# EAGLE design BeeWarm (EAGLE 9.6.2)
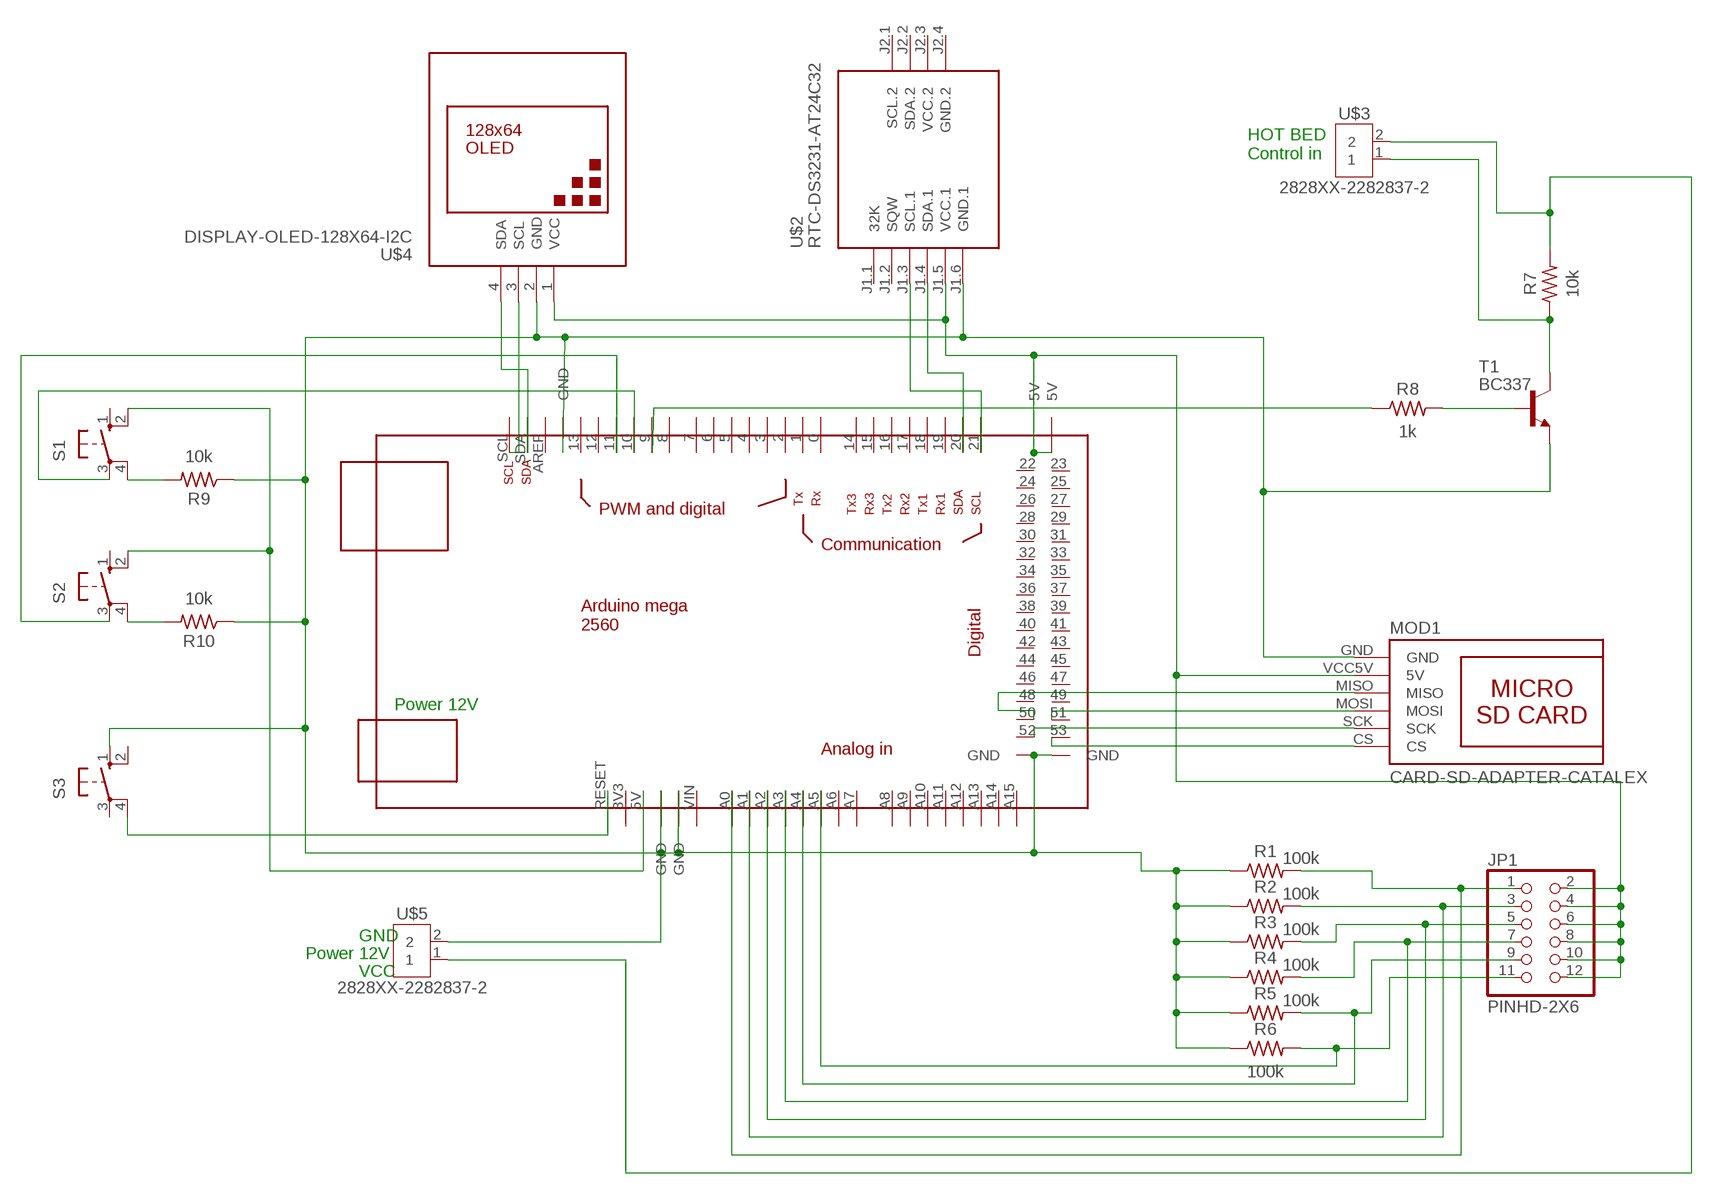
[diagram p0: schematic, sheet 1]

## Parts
JP1  PINHD-2X6  [2X06]
MOD1  CARD-SD-ADAPTER-CATALEX  [CARD-SD-ADAPTER-CATALEX]
R1  100k  R-US_AXIAL-11.7MM-PITCH  [RESAD1176W63L850D250B]
R2  100k  R-US_AXIAL-11.7MM-PITCH  [RESAD1176W63L850D250B]
R3  100k  R-US_AXIAL-11.7MM-PITCH  [RESAD1176W63L850D250B]
R4  100k  R-US_AXIAL-11.7MM-PITCH  [RESAD1176W63L850D250B]
R5  100k  R-US_AXIAL-11.7MM-PITCH  [RESAD1176W63L850D250B]
R6  100k  R-US_AXIAL-11.7MM-PITCH  [RESAD1176W63L850D250B]
R7  10k  R-US_AXIAL-11.7MM-PITCH  [RESAD1176W63L850D250B]
R8  1k  R-US_AXIAL-11.7MM-PITCH  [RESAD1176W63L850D250B]
R9  10k  R-US_AXIAL-11.7MM-PITCH  [RESAD1176W63L850D250B]
R10  10k  R-US_AXIAL-11.7MM-PITCH  [RESAD1176W63L850D250B]
S1  10-XX  [B3F-10XX]
S2  10-XX  [B3F-10XX]
S3  10-XX  [B3F-10XX]
T1  BC337  [TO92]
U$1  MEGA_DEVICE  [MEGAOUTLINE]
U$2  RTC-DS3231-AT24C32  [RTC-DS3231-AT24C32]
U$3  2828XX-2282837-2  [TERMBLK_508-2N]
U$4  DISPLAY-OLED-128X64-I2C  [DISPLAY-OLED-128X64-I2C]
U$5  2828XX-2282837-2  [TERMBLK_508-2N]

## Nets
N$2: S3.4(P1) U$1.RESET
N$3: MOD1.GND R1.1 R2.1 R3.1 R4.1 R5.1 R6.1 R9.1 R10.1 S3.1(S) T1.1(E) U$1.GND@1(GND) U$1.GND@2(GND) U$1.GND@3(GND) U$1.GND@6(GND) U$1.GND@7(GND) U$2.J1.6(GND.1) U$4.2(GND) U$5.2
N$5: JP1.1 R1.2 U$1.A0
N$6: JP1.3 R2.2 U$1.A1
N$7: JP1.5 R3.2 U$1.A2
N$8: JP1.7 R4.2 U$1.A3
N$9: JP1.9 R5.2 U$1.A4
N$10: JP1.11 R6.2 U$1.A5
N$11: U$1.20 U$2.J1.4(SDA.1)
N$12: U$1.21 U$2.J1.3(SCL.1)
N$13: U$1.SDA U$4.4(SDA)
N$14: MOD1.MOSI U$1.51
N$15: MOD1.SCK U$1.52
N$16: MOD1.CS U$1.53
N$17: MOD1.MISO U$1.50
N$18: U$1.SCL U$4.3(SCL)
N$19: R8.2 T1.2(B)
N$20: R7.1 T1.3(C) U$3.1
N$21: R7.2 U$3.2 U$5.1
N$22: R9.2 S1.4(P1)
N$23: R8.1 U$1.9
N$24: R10.2 S2.4(P1)
N$25: S1.3(P) U$1.10
N$26: S2.3(P) U$1.11
N$27: S1.2(S1) S2.2(S1) U$1.5V
N$29: JP1.2 JP1.4 JP1.6 JP1.8 JP1.10 JP1.12 MOD1.VCC5V(5V) U$1.GND@4(5V) U$1.GND@5(5V) U$2.J1.5(VCC.1) U$4.1(VCC)
Unconnected: S1.1(S) S2.1(S) S3.2(S1) S3.3(P) U$1.0 U$1.1 U$1.2 U$1.3 U$1.3V3 U$1.4 U$1.5 U$1.6 U$1.7 U$1.8 U$1.12 U$1.13 U$1.14 U$1.15 U$1.16 U$1.17 U$1.18 U$1.19 U$1.22 U$1.23 U$1.24 U$1.25 U$1.26 U$1.27 U$1.28 U$1.29 U$1.30 U$1.31 U$1.32 U$1.33 U$1.34 U$1.35 U$1.36 U$1.37 U$1.38 U$1.39 U$1.40 U$1.41 U$1.42 U$1.43 U$1.44 U$1.45 U$1.46 U$1.47 U$1.48 U$1.49 U$1.A6 U$1.A7 U$1.A8 U$1.A9 U$1.A10 U$1.A11 U$1.A12 U$1.A13 U$1.A14 U$1.A15 U$1.AREF U$1.VIN U$2.J1.1(32K) U$2.J1.2(SQW) U$2.J2.1(SCL.2) U$2.J2.2(SDA.2)

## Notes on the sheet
- HOT BED 
  Control in
- Power 12V
- GND
- Power 12V
- VCC

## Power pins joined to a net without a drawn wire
GND.2: U$2.J2.4(GND.2)
VCC.2: U$2.J2.3(VCC.2)

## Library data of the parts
JP1 = Connector:PINHD-2X6: PIN HEADER; CATEGORY: CONNECTOR; SUB-CATEGORY: PIN-HEADER
MOD1 = SD-Card-Module_CATALEX:CARD-SD-ADAPTER-CATALEX: Micro SD Card Adapter Module with onboard 3.3V regulator
R1-R10 = Resistor:R-US: Resistor Fixed - ANSI; CATEGORY: Resistor; SUB-CATEGORY: Fixed
S1-S3 = switch-omron:10-XX: OMRON SWITCH; MPN: B3F-1000; OC_FARNELL: 176432; OC_NEWARK: 36M3542
T1 = transistor:BC337: NPN TRANSISTOR
U$1 = ArduinoMegaOutline:MEGA_DEVICE: mega card as device
U$2 = diy-modules:RTC-DS3231-AT24C32: RTC Module with Battery and EEPROM based on DS3231 and AT24C32 chips Tutorial can be found here: https://edwardmallon.wordpress.com/2014/05/21/using-a-cheap-3-ds3231-rtc-at24c32-eeprom-from-ebay/ Click here to find device on ebay.com
U$3 U$5 = Connector:2828XX-2: 2 Position Wire to Board Terminal Block Horizontal with Board; CATEGORY: Connector; DESCRIPTION: 2 Position Wire to Board Terminal Block Horizontal with Board 5.08 mm Through Hole; MANUFACTURER: TE Connectivity; MPN: 282837-2; OPERATING_TEMPERATURE: -40°C to +105°C; PART_STATUS: ACTIVE; ROHS_COMPLIANCE: RoHS Compliant; SERIES: 282837; SUBCATEGORY: Terminal Block; TYPE: Side Wire Entry
U$4 = diy-modules (1):DISPLAY-OLED-128X64-I2C: 128x64 Dot Matrix OLED Module based on SSD1306 chip Variant with I2C interface More details available here: http://www.instructables.com/id/Monochrome-096-i2c-OLED-display-with-arduino-SSD13/ SSD1306 datasheet: https://cdn-shop.adafruit.com/datasheets/SSD1306.pdf Click here to find device on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

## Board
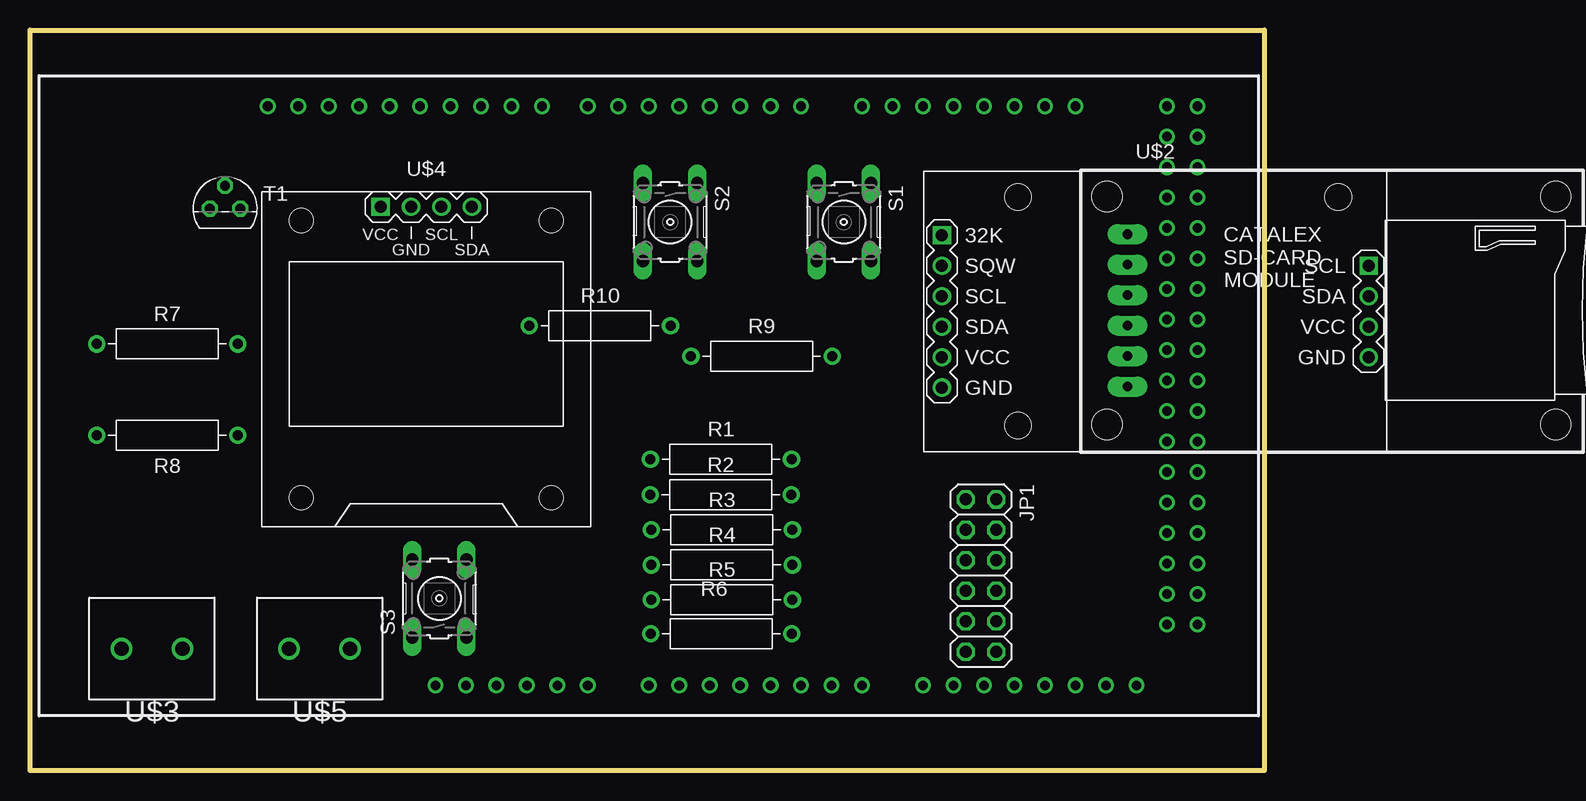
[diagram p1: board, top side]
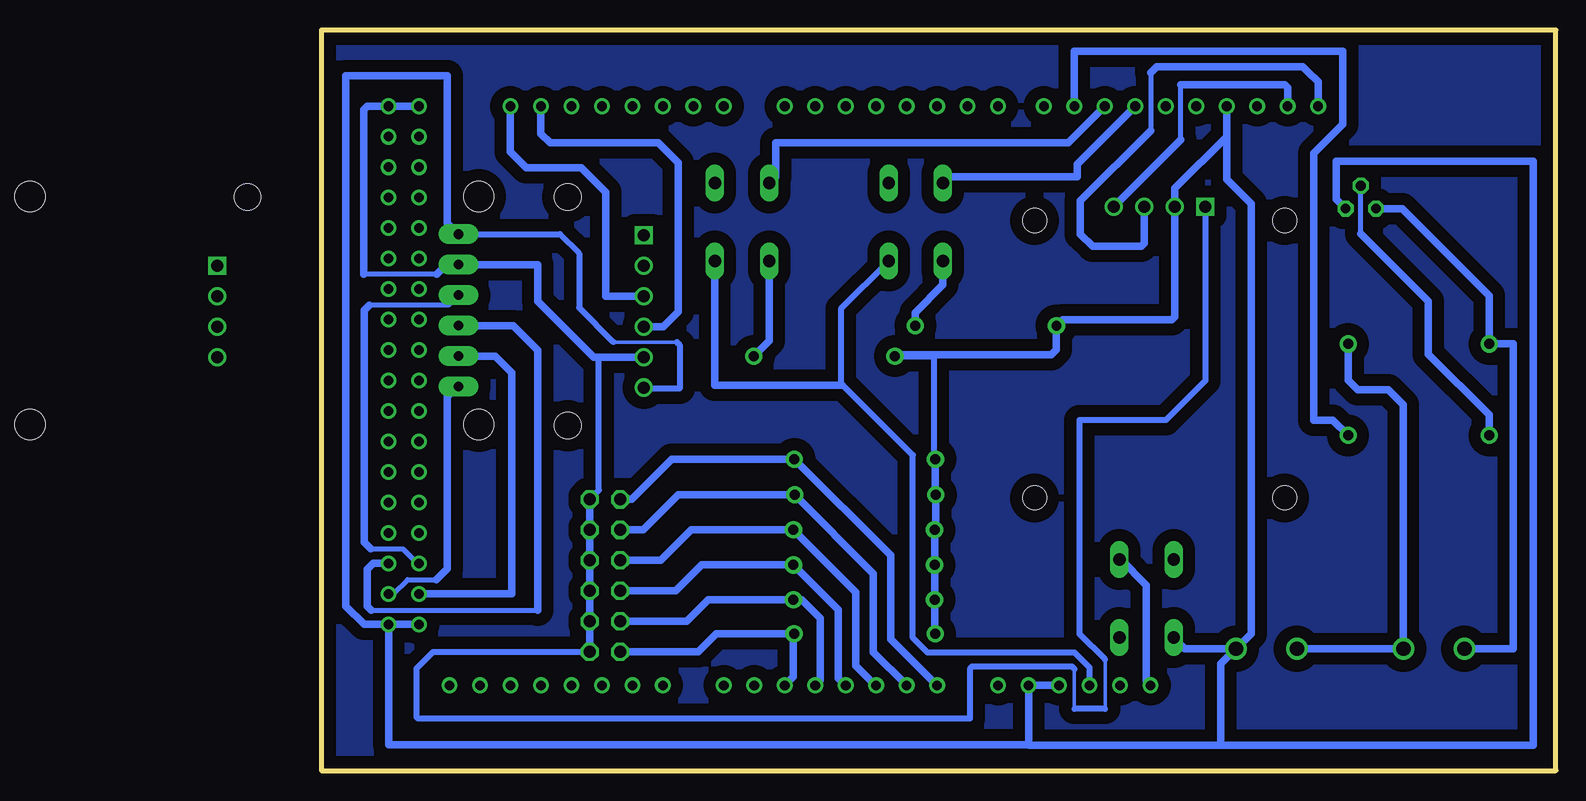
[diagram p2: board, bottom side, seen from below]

Size 102.87 x 61.72 mm. Coordinates in mm from the lower left corner, seen from the top.
Outline: 0,0 0,61.72 102.87,61.72 102.87,0 0,0
Copper layers (1*16): Top 0.035mm / dielectric 1.5mm / Bottom 0.035mm
Design rules "default": minimum track width 6mil, minimum drill 0.35mm, track to track 6mil, track to pad 6mil, pad to pad 6mil, via to via 6mil, smd to smd 6mil, copper to edge 40mil, drill to drill 6mil, minimum pad ring 10mil, minimum via ring 8mil, stop-mask expansion 4mil, vias tented up to drill 0mil, thermal gap 10mil

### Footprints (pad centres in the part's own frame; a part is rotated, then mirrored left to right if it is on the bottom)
2X06 = drill 1.016 octagon: 1 -6.35,-1.27; 2 -6.35,1.27; 3 -3.81,-1.27; 4 -3.81,1.27; 5 -1.27,-1.27; 6 -1.27,1.27; 7 1.27,-1.27; 8 1.27,1.27; 9 3.81,-1.27; 10 3.81,1.27; 11 6.35,-1.27; 12 6.35,1.27
CARD-SD-ADAPTER-CATALEX = drill 0.8 pad 1.676 long: CS -17,-6.35; GND -17,6.35; MISO -17,1.27; MOSI -17,-1.27; SCK -17,-3.81; VCC5V -17,3.81 | hole 2.5: -18.7,9.5; 18.7,9.5; 18.7,-9.5; -18.7,-9.5
RESAD1176W63L850D250B = drill 0.83 pad 1.43: 1 -5.88,0; 2 5.88,0
B3F-10XX = drill 1.016 long: 1 -3.251,2.261; 2 3.251,2.261; 3 -3.251,-2.261; 4 3.251,-2.261
TO92 = drill 0.813 octagon: 1 1.27,0; 2 0,1.905; 3 -1.27,0
MEGAOUTLINE = drill 0.8: 0 12.7,24.13; 1 10.16,24.13; 2 7.62,24.13; 3 5.08,24.13; 3V3 -15.24,-24.13; 4 2.54,24.13; 5 0,24.13; 5V -12.7,-24.13; 6 -2.54,24.13; 7 -5.08,24.13; 8 -8.89,24.13; 9 -11.43,24.13; 10 -13.97,24.13; 11 -16.51,24.13; 12 -19.05,24.13; 13 -21.59,24.13; 14 17.78,24.13; 15 20.32,24.13; 16 22.86,24.13; 17 25.4,24.13; 18 27.94,24.13; 19 30.48,24.13; 20 33.02,24.13; 21 35.56,24.13; 22 43.18,21.59; 23 45.72,21.59; 24 43.18,19.05; 25 45.72,19.05; 26 43.18,16.51; 27 45.72,16.51; 28 43.18,13.97; 29 45.72,13.97; 30 43.18,11.43; 31 45.72,11.43; 32 43.18,8.89; 33 45.72,8.89; 34 43.18,6.35; 35 45.72,6.35; 36 43.18,3.81; 37 45.72,3.81; 38 43.18,1.27; 39 45.72,1.27; 40 43.18,-1.27; 41 45.72,-1.27; 42 43.18,-3.81; 43 45.72,-3.81; 44 43.18,-6.35; 45 45.72,-6.35; 46 43.18,-8.89; 47 45.72,-8.89; 48 43.18,-11.43; 49 45.72,-11.43; 50 43.18,-13.97; 51 45.72,-13.97; 52 43.18,-16.51; 53 45.72,-16.51; A0 0,-24.13; A1 2.54,-24.13; A2 5.08,-24.13; A3 7.62,-24.13; A4 10.16,-24.13; A5 12.7,-24.13; A6 15.24,-24.13; A7 17.78,-24.13; A8 22.86,-24.13; A9 25.4,-24.13; A10 27.94,-24.13; A11 30.48,-24.13; A12 33.02,-24.13; A13 35.56,-24.13; A14 38.1,-24.13; A15 40.64,-24.13; AREF -26.67,24.13; GND@1 -24.13,24.13; GND@2 -10.16,-24.13; GND@3 -7.62,-24.13; GND@4 43.18,24.13; GND@5 45.72,24.13; GND@6 43.18,-19.05; GND@7 45.72,-19.05; RESET -17.78,-24.13; SCL -31.75,24.13; SDA -29.21,24.13; VIN -5.08,-24.13
RTC-DS3231-AT24C32 = drill 1 square: J1.1 -17.78,6.35; J2.1 17.78,3.81 | drill 1: J1.2 -17.78,3.81; J1.3 -17.78,1.27; J1.4 -17.78,-1.27; J1.5 -17.78,-3.81; J1.6 -17.78,-6.35; J2.2 17.78,1.27; J2.3 17.78,-1.27; J2.4 17.78,-3.81 | hole 2.2: -11.43,-9.525; -11.43,9.525; 15.24,9.525
TERMBLK_508-2N = drill 1.2: 1 0,0; 2 5.08,0
DISPLAY-OLED-128X64-I2C = drill 1 square: 1 -3.81,12.7 | drill 1: 2 -1.27,12.7; 3 1.27,12.7; 4 3.81,12.7 | hole 2: -10.414,11.557; 10.414,11.557; 10.414,-11.557; -10.414,-11.557

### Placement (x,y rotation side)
JP1  79.25,16.26 270 top
MOD1  108.46,38.35 0 top
R1  57.58,25.96 0 top
R2  57.56,22.99 0 top
R3  57.66,20.07 0 top
R4  57.66,17.14 0 top
R5  57.66,14.25 0 top
R6  57.61,11.4 0 top
R7  11.43,35.56 0 top
R8  11.43,27.94 180 top
R9  60.96,34.54 0 top
R10  47.5,37.08 0 top
S1  67.82,45.72 270 top
S2  53.34,45.72 270 top
S3  34.11,14.35 90 top
T1  16.26,46.84 0 top
U$1  51.56,31.24 0 top
U$2  93.78,38.28 0 top
U$3  7.62,10.16 0 top
U$4  33.02,34.29 0 top
U$5  21.59,10.16 0 top

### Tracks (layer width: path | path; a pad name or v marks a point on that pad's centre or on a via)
N$1
  pour Bottom (isolate 1.016): 0.08,61.82 102.69,61.82 102.84,61.67 102.84,0.08 0,0 0,61.67 0.08,61.75
N$2
  Bottom 0.152: 36.27,17.6 S3.4
  Bottom 0.61: U$1.RESET 34.14,7.47 34.14,15.47 36.27,17.6
N$3
  Bottom 0.305: 78.54,35.71 73.25,35.71
  Bottom 0.406: U$1.GND@3 43.94,2.13 | 27.43,52.83 U$1.GND@1 | R4.1 R5.1
  Bottom 0.508: R1.1 51.85,26.11 51.85,34.54 R9.1 | MOD1.GND 83.01,44.7 81.41,43.1 81.41,38.58 78.54,35.71 | 73.25,35.71 73.03,35.48 73.03,31.83 75.89,31.83 U$2.J1.6
  Bottom 0.61: 27.94,2.13 1.88,2.13 1.88,50.8 18.29,50.8 18.29,47.6 T1.1 | 43.94,2.13 27.94,2.13 | U$1.GND@2 U$1.GND@3 43.94,2.16 97.28,2.16 U$1.GND@7 | U$5.2 27.94,8.89 27.94,2.13 | R9.1 54.95,34.67 42.04,34.67 41.62,35.09 R10.1 41.11,37.59 32,37.59 31.75,37.85 U$4.2 31.75,48.51 27.43,52.83 | U$1.GND@1 27.43,49.28 25.4,47.24 25.4,11.43 U$5.2 | U$1.GND@7 99.31,12.19 100.84,13.72 100.84,57.91 92.38,57.91 92.38,45.63 MOD1.GND | U$1.GND@7 U$1.GND@6 | U$5.2 30.91,10.16 S3.1 | R1.1 51.7,23.01 R2.1 51.68,20.17 R3.1 R4.1 51.78,11.46 R6.1
N$5
  Bottom 0.61: JP1.1 77.01,22.61 73.66,25.96 R1.2 55.45,17.95 55.45,10.95 51.61,7.11 U$1.A0
N$6
  Bottom 0.61: JP1.3 76.07,20.07 73.15,22.99 R2.2 56.87,16.42 56.87,9.88 U$1.A1
N$7
  Bottom 0.61: JP1.5 74.6,17.53 72.06,20.07 R3.2 58.34,14.87 58.34,8.74 56.72,7.11 U$1.A2
N$8
  Bottom 0.61: JP1.7 73.33,14.99 71.17,17.14 R4.2 59.82,13.42 59.82,7.7 59.23,7.11 U$1.A3
N$9
  Bottom 0.61: JP1.9 72.44,12.45 70.64,14.25 R5.2 62.85,14.25 61.32,12.71 61.32,7.52 U$1.A4
N$10
  Bottom 0.61: JP1.11 71.48,9.91 69.98,11.4 R6.2 63.56,11.33 63.56,7.81 U$1.A5
N$11
  Bottom 0.61: U$1.20 84.58,53.09 83.82,52.32 74.8,52.32 73.13,50.65 73.13,38.25 74.37,37.01 U$2.J1.4
N$12
  Bottom 0.61: U$2.J1.3 79.2,39.55 79.2,48.21 81.23,50.24 85.8,50.24 87.12,51.56 U$1.21
N$13
  Bottom 0.406: 31.24,52.58 31.24,57.15
  Bottom 0.61: U$4.4 31.24,52.58 | 31.24,57.15 22.61,57.15 22.35,56.9 U$1.SDA
N$14
  Bottom 0.406: 98.73,13.39 84.84,13.39
  Bottom 0.61: U$1.51 98.55,17.27 99.06,16.76 99.06,13.72 98.73,13.39 | 84.84,13.39 84.84,35.05 86.87,37.08 MOD1.MOSI
N$15
  Bottom 0.61: U$1.52 87.02,14.73 87.02,33.17 88.39,34.54 MOD1.SCK
N$16
  Bottom 0.406: U$1.53 96.88,14.73 95.68,15.93 93.29,15.93
  Bottom 0.61: MOD1.CS 91.57,32 92.41,31.17 92.41,16.82 93.29,15.93
N$17
  Bottom 0.406: MOD1.MISO 92.3,38.79 98.88,38.79 | 98.75,18.49 96.09,18.49 94.87,17.27 U$1.50
  Bottom 0.61: 98.88,38.79 99.31,38.35 99.31,19.05 98.75,18.49
N$18
  Bottom 0.406: 33.78,58.17 33.78,53.34 | 20.7,58.29
  Bottom 0.61: U$1.SCL 19.81,57.4 20.7,58.29 21.08,58.67 33.27,58.67 33.78,58.17 | U$4.3 34.29,43.94 34.54,43.69 38.61,43.69 39.62,44.7 39.62,47.5 33.78,53.34
N$19
  Bottom 0.406: 16.26,44.76 T1.2
  Bottom 0.61: R8.2 5.55,29.66 10.62,34.72 10.62,39.12 16.26,44.76
N$20
  Bottom 0.61: U$3.1 3.56,10.16 3.56,35.56 R7.1 5.55,39.59 12.8,46.84 T1.3
N$21
  Bottom 0.61: R7.2 17.31,32.55 16.51,31.75 13.97,31.75 12.7,30.48 U$3.2 U$5.1
N$22
  Bottom 0.61: R9.2 65.56,35.83 S1.4
N$23
  Bottom 0.61: R8.1 18.58,29.21 20.19,29.21 20.19,51.46 17.78,53.87 17.78,59.94 40.13,59.94 U$1.9
N$24
  Bottom 0.61: R10.2 53.38,38.18 51.08,40.48 S2.4
N$25
  Bottom 0.61: S1.3 65.02,49.51 65.02,52.32 40.64,52.32 U$1.10
N$26
  Bottom 0.61: U$1.11 39.88,50.55 39.88,49.48 50.57,49.48 S2.3
N$27
  Bottom 0.508: S2.2 59.59,38.48 59.59,32.12 | U$1.5V 38.86,8.59 40.11,9.83 52.35,9.83 53.59,11.07 53.59,26.29 59.42,32.12 66.73,32.12
  Bottom 0.61: 59.59,32.12 66.73,32.12 70.08,32.12 S1.2
N$29
  Bottom 0.305: 37.57,9.27 37.57,5.16 | 40.13,5.16 40.13,8.48
  Bottom 0.406: JP1.2 JP1.4 | JP1.10 JP1.8 JP1.6 | 93.27,41.35 99.36,41.35
  Bottom 0.508: JP1.2 79.76,23.37 79.76,34.47 | U$4.1 29.21,32.51 32.51,29.21 39.7,29.21 39.7,11.4 37.57,9.27 | 37.57,5.16 40.13,5.16 | 40.13,8.48 40.31,8.66 48.67,8.66 48.84,8.48 48.84,4.34 94.82,4.34 94.94,4.47 94.94,8.53 93.57,9.91 JP1.12
  Bottom 0.61: JP1.12 JP1.10 JP1.6 JP1.2 | U$2.J1.5 79.76,34.47 80.19,34.47 84.84,39.12 84.84,42.16 MOD1.VCC5V 92.46,42.16 93.27,41.35 | U$1.GND@4 U$1.GND@5 99.06,55.37 99.36,55.07 99.36,41.35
